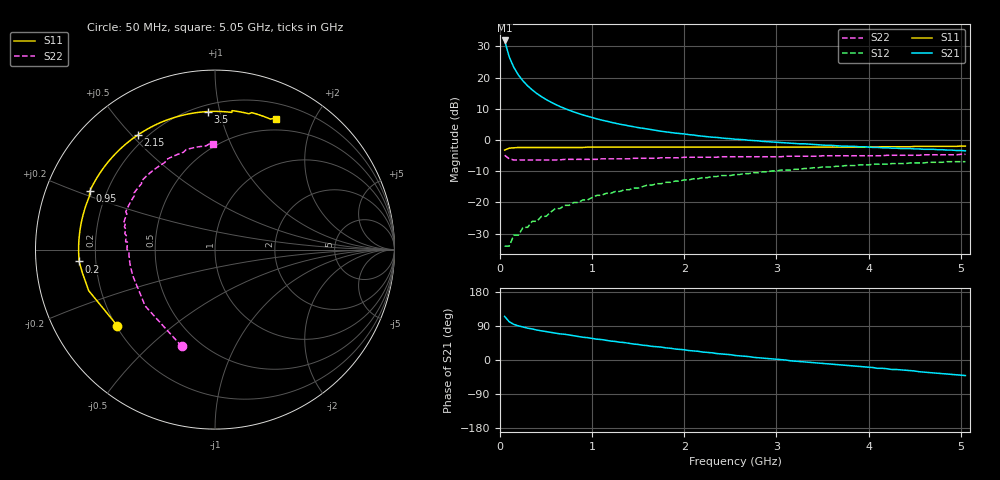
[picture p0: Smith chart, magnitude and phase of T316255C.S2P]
!AT-31625
!S-PARAMETERS at Vce=4.8 V  Ic=150 mA.  LAST UPDATED 08-05-96
# ghz s ma r 50
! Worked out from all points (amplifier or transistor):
!   101 points, 50 MHz to 5.05 GHz, reference 50 ohm
!   highest |S21| = 31.9 dB at 50 MHz (marker M1)
!   |S21| within 3 dB of that: start of sweep to 78.59 MHz
!   unconditionally stable (mu >= 1): 399.5647 MHz to 401.3407 MHz; 469.1 MHz to 1.549 GHz; 1.74995 GHz to 1.750028 GHz
!   at 850 MHz: K = 1.06, MAG = 12.8 dB, |S12| = -20.0 dB
!   at 2.55 GHz: K = 0.96, MSG = 5.7 dB, |S12| = -11.1 dB
!   at 5.05 GHz: K = 0.94, MSG = 1.7 dB, |S12| = -6.9 dB
!   S11 on the Smith chart (normalised r, x): 50 MHz: 0.20, -0.33; 200 MHz: 0.14, -0.04; 950 MHz: 0.14, +0.22; 2.15 GHz: 0.17, +0.52; 3.5 GHz: 0.24, +0.92; 5.05 GHz: 0.37, +1.50
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0.05  0.69 -142.0  39.19 115.0  0.02 42.0  0.57 -109.0
0.1  0.74 -162.0  21.42 101.0  0.02 42.0  0.5 -141.0
0.15  0.75 -170.0  14.52 94.0  0.03 48.0  0.48 -154.0
0.2  0.76 -175.0  10.96 90.0  0.03 52.0  0.48 -161.0
0.25  0.76 -179.0  8.81 87.0  0.04 56.0  0.48 -165.0
0.3  0.76 178.0  7.36 84.0  0.04 58.0  0.48 -168.0
0.35  0.76 176.0  6.33 82.0  0.05 60.0  0.48 -170.0
0.4  0.76 174.0  5.54 79.0  0.05 62.0  0.48 -172.0
0.5  0.76 170.0  4.45 75.0  0.06 63.0  0.48 -175.0
0.6  0.76 166.0  3.72 71.0  0.08 64.0  0.48 -178.0
0.75  0.76 162.0  3 66.0  0.09 63.0  0.49 180.0
0.9  0.76 157.0  2.52 60.0  0.11 62.0  0.49 177.0
0.95  0.77 155.0  2.4 59.0  0.11 62.0  0.49 177.0
1.05  0.77 153.0  2.18 55.0  0.13 60.0  0.49 175.0
1.3  0.77 146.0  1.79 47.0  0.15 57.0  0.5 172.0
1.75  0.77 134.0  1.38 34.0  0.2 50.0  0.52 166.0
2.15  0.77 124.0  1.17 23.0  0.24 43.0  0.53 161.0
2.55  0.77 114.0  1.03 12.0  0.28 36.0  0.54 155.0
3.4  0.77 95.0  0.85 -7.0  0.36 21.0  0.55 139.0
3.5  0.77 93.0  0.83 -9.0  0.37 19.0  0.56 137.0
4.25  0.78 79.0  0.74 -25.0  0.42 3.0  0.57 117.0
5.05  0.8 65.0  0.67 -41.0  0.45 -14.0  0.59 91.0
